(* Logix 5000 AddOnInstructionDefinition export DXM_Sign_Fix; software revision 30.00 *)

TYPE DXM_UDT :
STRUCT
   DTI : INT[228];   // Data that will be converted
   Data : DINT[228];   // Converted Data.
   Exception : SINT[48];   // Exclude input tag.
END_STRUCT
END_TYPE

ADD_ON_INSTRUCTION DXM_Sign_Fix   (* revision 2.0, vendor Banner Engineering *)
// DXM data is moved from INT to DINT to allow for 0 to 65535.
VAR_IN_OUT
   DXM : DXM_UDT; {required}
END_VAR
VAR_INPUT
   Num_Nodes : DINT := 1; {required}
END_VAR
VAR
   Index : INT; {access None}
   N_Index : INT; {access None}
   Control : DINT; {access None}
END_VAR

ROUTINE Logic   (* ladder *)
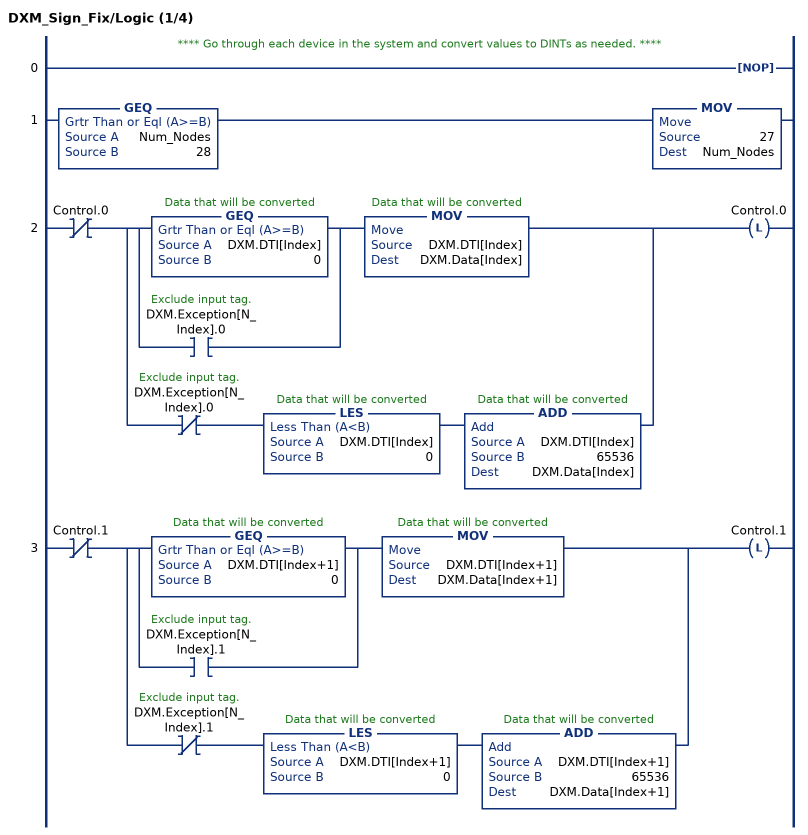
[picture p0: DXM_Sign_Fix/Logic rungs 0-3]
   // **** Go through each device in the system and convert values to DINTs as needed. ****
   0: NOP();
   1: GEQ(Num_Nodes,28)MOV(27,Num_Nodes);
   2: XIO(Control.0)[[GEQ(DXM.DTI[Index],0) ,XIC(DXM.Exception[N_Index].0) ] MOV(DXM.DTI[Index],DXM.Data[Index]) ,XIO(DXM.Exception[N_Index].0) LES(DXM.DTI[Index],0) ADD(DXM.DTI[Index],65536,DXM.Data[Index]) ]OTL(Control.0);
   3: XIO(Control.1)[[GEQ(DXM.DTI[Index+1],0) ,XIC(DXM.Exception[N_Index].1) ] MOV(DXM.DTI[Index+1],DXM.Data[Index+1]) ,XIO(DXM.Exception[N_Index].1) LES(DXM.DTI[Index+1],0) ADD(DXM.DTI[Index+1],65536,DXM.Data[Index+1]) ]OTL(Control.1);
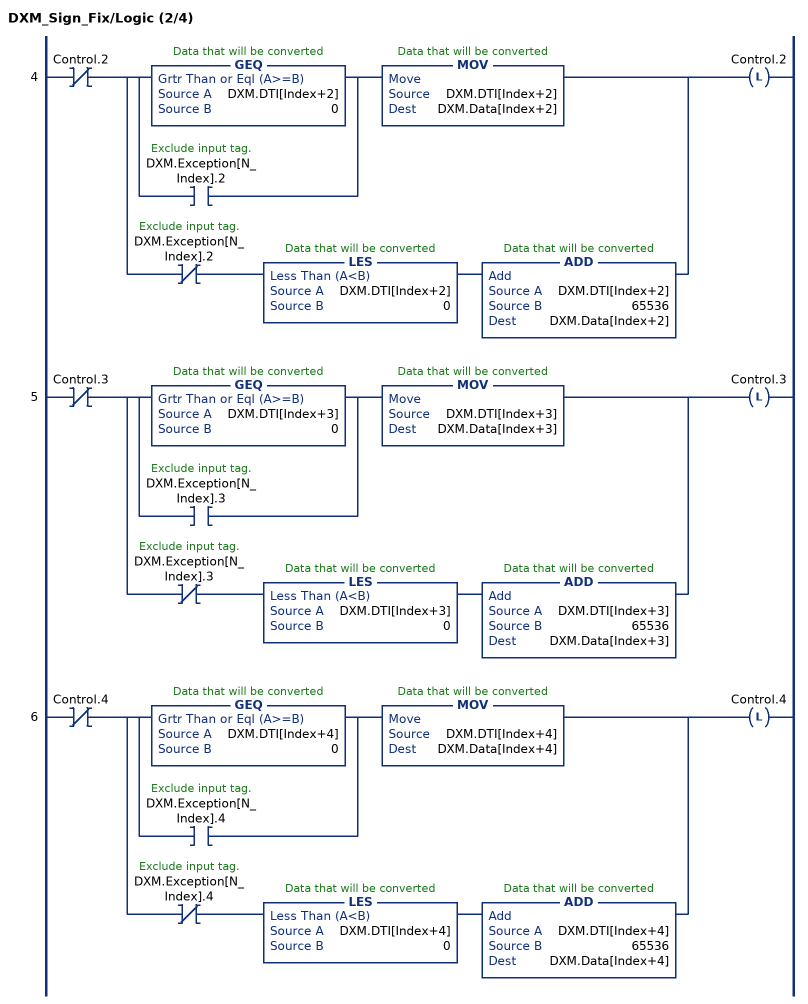
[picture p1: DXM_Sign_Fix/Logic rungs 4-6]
   4: XIO(Control.2)[[GEQ(DXM.DTI[Index+2],0) ,XIC(DXM.Exception[N_Index].2) ] MOV(DXM.DTI[Index+2],DXM.Data[Index+2]) ,XIO(DXM.Exception[N_Index].2) LES(DXM.DTI[Index+2],0) ADD(DXM.DTI[Index+2],65536,DXM.Data[Index+2]) ]OTL(Control.2);
   5: XIO(Control.3)[[GEQ(DXM.DTI[Index+3],0) ,XIC(DXM.Exception[N_Index].3) ] MOV(DXM.DTI[Index+3],DXM.Data[Index+3]) ,XIO(DXM.Exception[N_Index].3) LES(DXM.DTI[Index+3],0) ADD(DXM.DTI[Index+3],65536,DXM.Data[Index+3]) ]OTL(Control.3);
   6: XIO(Control.4)[[GEQ(DXM.DTI[Index+4],0) ,XIC(DXM.Exception[N_Index].4) ] MOV(DXM.DTI[Index+4],DXM.Data[Index+4]) ,XIO(DXM.Exception[N_Index].4) LES(DXM.DTI[Index+4],0) ADD(DXM.DTI[Index+4],65536,DXM.Data[Index+4]) ]OTL(Control.4);
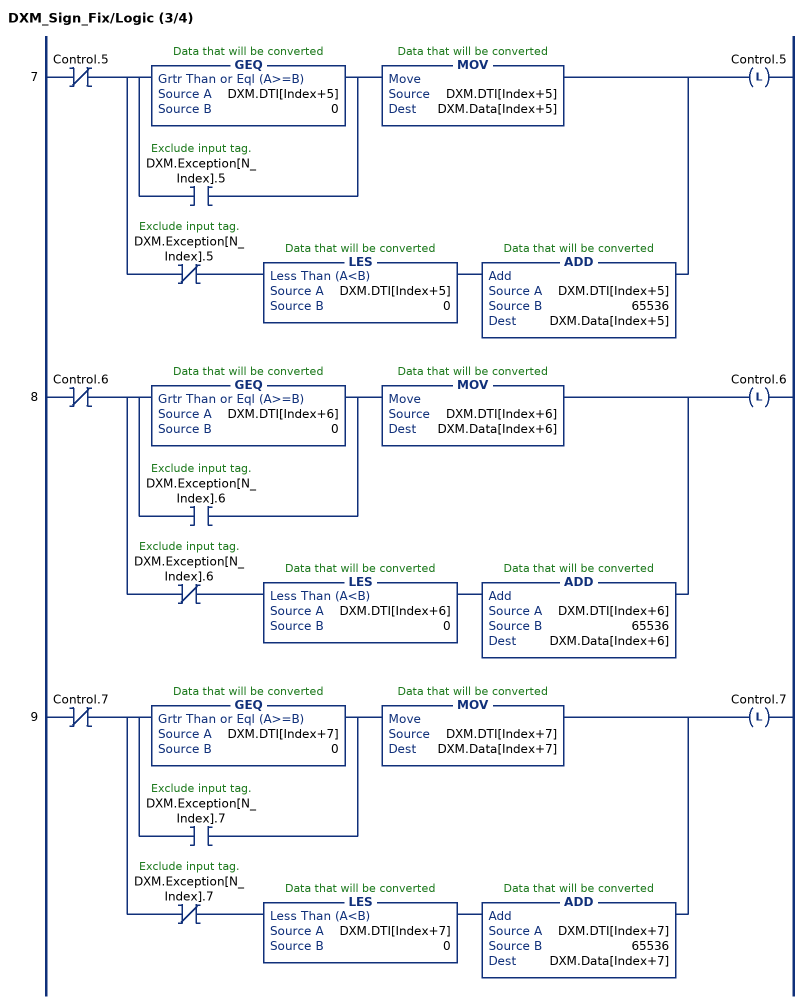
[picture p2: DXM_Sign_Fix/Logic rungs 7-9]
   7: XIO(Control.5)[[GEQ(DXM.DTI[Index+5],0) ,XIC(DXM.Exception[N_Index].5) ] MOV(DXM.DTI[Index+5],DXM.Data[Index+5]) ,XIO(DXM.Exception[N_Index].5) LES(DXM.DTI[Index+5],0) ADD(DXM.DTI[Index+5],65536,DXM.Data[Index+5]) ]OTL(Control.5);
   8: XIO(Control.6)[[GEQ(DXM.DTI[Index+6],0) ,XIC(DXM.Exception[N_Index].6) ] MOV(DXM.DTI[Index+6],DXM.Data[Index+6]) ,XIO(DXM.Exception[N_Index].6) LES(DXM.DTI[Index+6],0) ADD(DXM.DTI[Index+6],65536,DXM.Data[Index+6]) ]OTL(Control.6);
   9: XIO(Control.7)[[GEQ(DXM.DTI[Index+7],0) ,XIC(DXM.Exception[N_Index].7) ] MOV(DXM.DTI[Index+7],DXM.Data[Index+7]) ,XIO(DXM.Exception[N_Index].7) LES(DXM.DTI[Index+7],0) ADD(DXM.DTI[Index+7],65536,DXM.Data[Index+7]) ]OTL(Control.7);
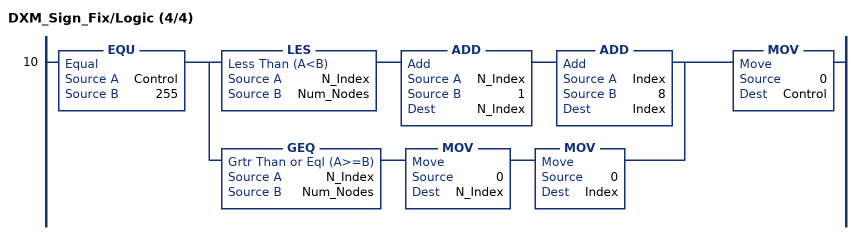
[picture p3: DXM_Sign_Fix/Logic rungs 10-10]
   10: EQU(Control,255)[LES(N_Index,Num_Nodes) ADD(N_Index,1,N_Index) ADD(Index,8,Index) ,GEQ(N_Index,Num_Nodes) MOV(0,N_Index) MOV(0,Index) ]MOV(0,Control);
END_ROUTINE
END_ADD_ON_INSTRUCTION
